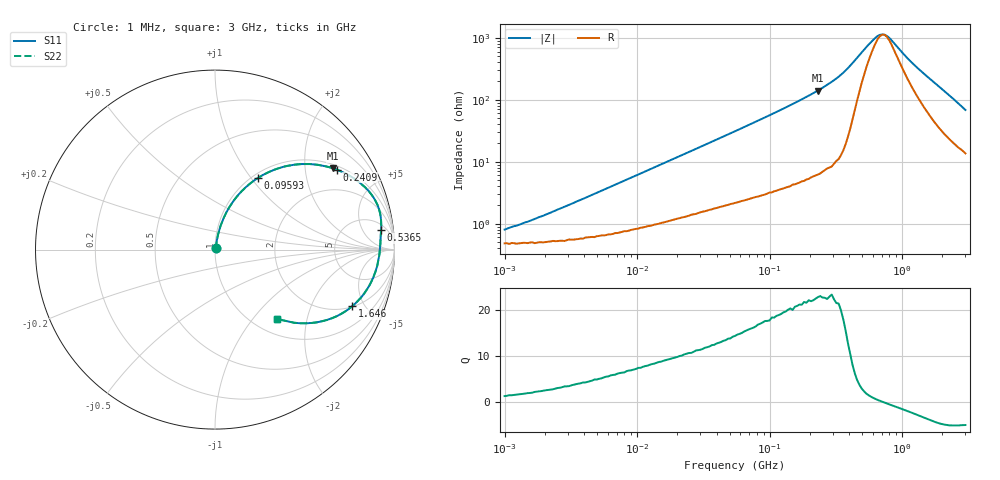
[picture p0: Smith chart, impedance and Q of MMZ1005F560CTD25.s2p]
! S-Parameter Data Generated by TDK Corporation
! Copyright(C) 2025 TDK Corporation.
! All Rights Reserved.
! TDK P/N: MMZ1005F560CTD25 (Chip Bead)
! Property: |Z|=56ohm at 100MHz
! Size(LxWxT): 1x0.5x0.5mm
! Model Type: s2p (Touchstone File Format Version 1.0)
! Frequency: DC=Yes Start=1MHz Stop=3000MHz 202points Log-sweep
! Model Generated on Feb. 6, 2025
! Terms and conditions regarding TDK Simulation Models:
! 1)This simulation model is being provided solely for informational
!  purposes. Please refer to the specifications of the products in
!  terms of detailed characteristics of such products.
! 2)In no event shall TDK Corporation of any of its subsidiaries be
!  liable for any loss or damage arising, directly or indirectly,
!  from any information contained in this simulation model, including,
!  but not limited to loss or damages arising from any inaccuracies,
!  omissions or errors in connection with such information.
! 3)Any and all copyrights on this simulation model are owned by
!  TDK Corporation.  Duplication or redistribution of this simulation
!  model without prior written permission from TDK Corporation
!  is prohibited.
! 4)This simulation model is subject to any modification or change
!  without any prior notice.
! 5)Neither TDK Corporation nor any of its subsidiaries shall make any
!  warranty, express or implied, including but not limited to the
!  correctness, implied warranties of merchantability and fitness for
!  a particular purpose with respect to this simulation models.
! 6)The use of this simulation model shall be deemed to have consented
!  to the terms and conditions hereof.
! Port Assignments:
!  1 ---@@@--- 2
! Applicable Conditions:
!  Temperature = 25 degC
!  DC Bias Current = 0 A
!  Small Signal Operation
# Hz S MA R 50
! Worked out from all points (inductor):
!   201 points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, 1 MHz to 3 GHz, reference 50 ohm
!   read as one part in series: L = 101 nH near 2.511 MHz
!   highest Q = 22.6 at 231.4 MHz (marker M1), where L = 96.7 nH
!   self-resonance near 725.5 MHz
!   S11 on the Smith chart (normalised r, x): 1 MHz: 1.01, +0.01; 95.93 MHz: 1.06, +1.08; 240.9 MHz: 1.13, +2.96; 536.5 MHz: 8, +12; 1.646 GHz: 2.05, -4.08; 3 GHz: 1.27, -1.34
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1000000  0.008005 52.9  0.9952 -0.4  0.9952 -0.4  0.008005 52.9
1682724  0.01178 65.2  0.9951 -0.6  0.9951 -0.6  0.01178 65.2
3900413  0.02498 75.4  0.994 -1.4  0.994 -1.4  0.02498 75.4
1.461624e7  0.08625 78.5  0.9865 -4.9  0.9865 -4.9  0.08625 78.5
3.00453e7  0.1687 75.3  0.971 -9.7  0.971 -9.7  0.1687 75.3
5.477226e7  0.2906 69.2  0.9368 -16.8  0.9368 -16.8  0.2906 69.2
9.593103e7  0.4639 59.1  0.8599 -27.6  0.8599 -27.6  0.4639 59.1
1.431579e8  0.6174 49.1  0.7568 -38.1  0.7568 -38.1  0.6174 49.1
2.136344e8  0.7706 37.1  0.6033 -50.3  0.6033 -50.3  0.7706 37.1
2.314421e8  0.7989 34.5  0.5673 -53.0  0.5673 -53.0  0.7989 34.5
2.408952e8  0.8125 33.2  0.5486 -54.3  0.5486 -54.3  0.8125 33.2
3.594878e8  0.9222 19.8  0.3386 -67.0  0.3386 -67.0  0.9222 19.8
4.391493e8  0.9418 12.5  0.2187 -68.4  0.2187 -68.4  0.9418 12.5
5.364635e8  0.931 6.7  0.1319 -55.2  0.1319 -55.2  0.931 6.7
6.296259e8  0.9236 3.1  0.09207 -32.4  0.09207 -32.4  0.9236 3.1
6.821091e8  0.9206 1.3  0.08252 -15.2  0.08252 -15.2  0.9206 1.3
7.38967e8  0.9181 -0.4  0.08218 4.6  0.08218 4.6  0.9181 -0.4
8.005644e8  0.9155 -2.2  0.09213 22.3  0.09213 22.3  0.9155 -2.2
1.147801e9  0.8916 -11.0  0.2108 53.7  0.2108 53.7  0.8916 -11.0
1.645649e9  0.8275 -22.4  0.3926 53.3  0.3926 53.3  0.8275 -22.4
2.266846e9  0.6976 -35.5  0.5923 43.2  0.5923 43.2  0.6976 -35.5
3e9  0.5181 -48.0  0.7582 30.5  0.7582 30.5  0.5181 -48.0
